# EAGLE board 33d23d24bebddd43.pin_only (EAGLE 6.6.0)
REV: B

Size 60.33 x 22.86 mm. Coordinates in mm from the lower left corner, seen from the top.
Outline: 2.54,0 57.78,0 arc90 60.33,2.54 60.33,20.32 arc90 57.78,22.86 2.54,22.86 arc90 0,20.32 0,14.1 0.51,13.59 0.51,9.4 0,8.89 0,2.54 arc90 2.54,0
Copper layers (1*16): Top 0.035mm / dielectric 1.5mm / Bottom 0.035mm
Design rules "adafruit 6-6 *": minimum track width 6mil, minimum drill 15.5mil, track to track 8mil, track to pad 6mil, pad to pad 8mil, via to via 8mil, smd to smd 8mil, copper to edge 10mil, drill to drill 8mil, minimum pad ring 10mil, minimum via ring 8mil, stop-mask expansion 2mil, vias tented up to drill 20mil, thermal gap 10mil
Holes 2.2 mm at 57.78,20.32
tRestrict: area 23.5,8.1 to 26.4,8.6; area 26.3,8.6 to 26.5,9.9; area 26.3,10.3 to 26.5,13.5; area 21,13.6 to 25.9,14; area 20.8,9.3 to 21.2,12.8; area 21.1,8.1 to 23,8.6; area 20.8,8.4 to 21.2,8.9; area 20.8,13.3 to 21.2,13.7

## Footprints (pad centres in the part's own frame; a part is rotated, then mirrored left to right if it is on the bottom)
_0805MP = smd 1.2 x 1.3: 1 -1.016,0; 2 1.016,0
0805-NO = smd 1.3 x 1.5: 1 -0.95,0; 2 0.95,0
C1210 = smd 1.6 x 2.7: 1 -1.4,0; 2 1.4,0
0603-NO = smd 1.1 x 1: 1 -0.85,0; 2 0.85,0
CHIPLED_0805_NOOUTLINE = smd 1.2 x 1.2: A 0,-1.05; C 0,1.05
SOD-323 = smd 1.35 x 0.8: A 1.27,0; C -1.27,0
SOT363 = smd 0.5 x 0.5: 1 -0.75,-0.9; 3 0.75,-0.9; 4 0.75,0.9; 6 -0.75,0.9 | smd 0.4 x 0.5: 2 0,-0.9; 5 0,0.9
SOD-123 = smd 1.4 x 1.4: A 1.85,0; C -1.85,0
TQFN44_7MM = smd 0.25 x 0.8: 1 -2.5,-3.475; 2 -2,-3.475; 3 -1.5,-3.475; 4 -1,-3.475; 5 -0.5,-3.475; 6 0,-3.475; 7 0.5,-3.475; 8 1,-3.475; 9 1.5,-3.475; 10 2,-3.475; 11 2.5,-3.475; 23 2.5,3.475; 24 2,3.475; 25 1.5,3.475; 26 1,3.475; 27 0.5,3.475; 28 0,3.475; 29 -0.5,3.475; 30 -1,3.475; 31 -1.5,3.475; 32 -2,3.475; 33 -2.5,3.475 | smd 0.8 x 0.25: 12 3.475,-2.5; 13 3.475,-2; 14 3.475,-1.5; 15 3.475,-1; 16 3.475,-0.5; 17 3.475,0; 18 3.475,0.5; 19 3.475,1; 20 3.475,1.5; 21 3.475,2; 22 3.475,2.5; 34 -3.475,2.5; 35 -3.475,2; 36 -3.475,1.5; 37 -3.475,1; 38 -3.475,0.5; 39 -3.475,0; 40 -3.475,-0.5; 41 -3.475,-1; 42 -3.475,-1.5; 43 -3.475,-2; 44 -3.475,-2.5 | smd 4.7 x 4.7: THERMAL 0,0
1X16_ROUND = drill 1 pad 1.676: 1 -19.05,0; 2 -16.51,0; 3 -13.97,0; 4 -11.43,0; 5 -8.89,0; 6 -6.35,0; 7 -3.81,0; 8 -1.27,0; 9 1.27,0; 10 3.81,0; 11 6.35,0; 12 8.89,0; 13 11.43,0; 14 13.97,0; 15 16.51,0; 16 19.05,0
1X12_ROUND = drill 1 pad 1.676: 1 -13.97,0; 2 -11.43,0; 3 -8.89,0; 4 -6.35,0; 5 -3.81,0; 6 -1.27,0; 7 1.27,0; 8 3.81,0; 9 6.35,0; 10 8.89,0; 11 11.43,0; 12 13.97,0
SOLDERJUMPER_CLOSEDWIRE = smd 1.168 x 1.6: 1 -0.762,0; 2 0.762,0 | smd 0.635 x 0.203: WIRE 0,0
KMR2 = smd 1 x 1: 1 2,0.8; 2 2,-0.8; 3 -2,0.8; 4 -2,-0.8
TESTPOINT_ROUND_1.5MM = smd 1.5 x 1.5: P$1 0,0
SIM800L = smd 1.1 x 0.9: 1 -8.1,5.6; 2 -8.1,4.2; 3 -8.1,2.8; 4 -8.1,1.4; 5 -8.1,0; 6 -8.1,-1.4; 7 -8.1,-2.8; 8 -8.1,-4.2; 9 -8.1,-5.6; 22 8.1,-5.6; 23 8.1,-4.2; 24 8.1,-2.8; 25 8.1,-1.4; 26 8.1,0; 27 8.1,1.4; 28 8.1,2.8; 29 8.1,4.2; 30 8.1,5.6; 43 -6.36,5.6; 44 -6.36,4.2; 45 -6.36,2.8; 46 -6.36,1.4; 47 -6.36,0; 48 -6.36,-1.4; 49 -6.36,-2.8; 50 -6.36,-4.2; 51 -6.36,-5.6; 60 6.36,-5.6; 61 6.36,-4.2; 62 6.36,-2.8; 63 6.36,-1.4; 64 6.36,0; 65 6.36,1.4; 66 6.36,2.8; 67 6.36,4.2; 68 6.36,5.6 | smd 0.9 x 1.1: 10 -7.7,-7.1; 11 -6.3,-7.1; 12 -4.9,-7.1; 13 -3.5,-7.1; 14 -2.1,-7.1; 15 -0.7,-7.1; 16 0.7,-7.1; 17 2.1,-7.1; 18 3.5,-7.1; 19 4.9,-7.1; 20 6.3,-7.1; 21 7.7,-7.1; 31 7.7,7.1; 32 6.3,7.1; 33 4.9,7.1; 34 3.5,7.1; 35 2.1,7.1; 36 0.7,7.1; 37 -0.7,7.1; 38 -2.1,7.1; 39 -3.5,7.1; 40 -4.9,7.1; 41 -6.3,7.1; 42 -7.7,7.1; 52 -4.9,-5.5; 53 -3.5,-5.5; 54 -2.1,-5.5; 55 -0.7,-5.5; 56 0.7,-5.5; 57 2.1,-5.5; 58 3.5,-5.5; 59 4.9,-5.5; 69 4.9,5.5; 70 3.5,5.5; 71 2.1,5.5; 72 0.7,5.5; 73 -0.7,5.5; 74 -2.1,5.5; 75 -3.5,5.5; 76 -4.9,5.5 | smd 1.5 x 1.5: 77 -3.9,3 | smd 2.3 x 2.7: 78 -3.9,0; 79 -3.9,-3; 80 -1.3,-3; 81 1.3,-3; 82 3.9,-3; 83 3.9,0; 84 3.9,3; 85 1.3,3; 86 -1.3,3; 87 -1.3,0; 88 1.3,0
SOT23-5 = smd 0.55 x 1.2: 1 -0.95,-1.3; 2 0,-1.3; 3 0.95,-1.3; 4 0.95,1.3; 5 -0.95,1.3
FIDUCIAL_1MM = smd 1 x 1: 1 0,0
MOUNTINGHOLE_2.5_PLATED = drill 2.5 pad 3.2: P$1 0,0
JSTPH2 = smd 1 x 4.6: 1 -1,-3.7; 2 1,-3.7 | smd 1.6 x 3.4: NC1 -3.4,1.5; NC2 3.4,1.5
4UCONN_20217 = smd 0.75 x 1.7: CLK -12.31,16.86; GND -5.96,16.86; I/O -11.04,16.86; RST -9.77,16.86; SW -4.69,16.86; VCC -7.23,16.86; VPP -8.5,16.86 | smd 1.4 x 1.05: GND@1 -15.53,17.06; GND@4 -0.33,17.06 | smd 1.5 x 2.7: GND@2 -15.86,1.42; GND@3 0,0
4UCONN_20329_V2 = smd 1 x 2: BASE@1 -0.75,-2; BASE@2 0.75,-2 | smd 0.4 x 1.35: D+ 0,0.775; D- -0.65,0.775; GND 1.3,0.775; ID 0.65,0.775; VBUS -1.3,0.775 | drill 0.8 pad 1.2 offset: SPRT@1 -3.3,0.9; SPRT@2 3.3,0.9 | drill 0.9 pad 2.5 square: SPRT@3 -3.6,-1.9; SPRT@4 3.6,-1.9 | hole 0.7: -1.95,0; 1.95,0
U.FL = smd 2.2 x 1.05: 1 0,1.375; 2 0,-1.375 | smd 0.8 x 1: 3 1.525,0
87758-0216 = drill 0.9 pad 1.27: 1 0,-1; 2 0,1
ANT_2450AT18B100 = smd 1.6 x 1.8: FP -1.4,0; NC 1.4,0
RESONATOR-SMD = smd 0.7 x 1.7: 1 -1.2,0; 2 0,0; 3 1.2,0

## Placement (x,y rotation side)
C1  10uF  [_0805MP]  37.27,9.02 180 top
C2  33pF  [0805-NO]  53.59,21.59 0 top
C3  10µF  [0805-NO]  11.81,12.06 0 top
C4  100uF  [C1210]  36.2,5.71 0 top
C5  10pF  [0805-NO]  50.16,21.59 180 top
C6  10µF  [0805-NO]  8.09,12.96 90 top
C7  1uF  [0603-NO]  18.94,15.04 90 top
C8  10µF  [0805-NO]  14.37,11.62 270 top
C9  10uF  [_0805MP]  29.57,15.46 180 top
C14  1uF  [0603-NO]  10.72,4.22 0 top
CHG  ORANGE  [CHIPLED_0805_NOOUTLINE]  2.41,5.59 270 top
D1  1N4148  [SOD-323]  33.78,12.32 270 top
D2  SMF05C  [SOT363]  37.47,12.19 0 top
D3  1N4148  [SOD-323]  32.77,17.4 270 top
D4  MBR120  [SOD-123]  17.91,18.92 180 top
D5  MMSZ5231BT1G  [SOD-123]  32.51,7.11 90 top
D7  1N4148  [SOD-323]  48.39,1.52 0 top
D9  1N4148  [SOD-323]  54.99,1.52 0 top
IC1  ATMEGA32U4-MU  [TQFN44_7MM]  23.72,11.1 0 top
JP1  [1X16_ROUND]  25.4,1.27 180 top
JP3  [1X12_ROUND]  30.48,21.59 0 top
L  RED  [CHIPLED_0805_NOOUTLINE]  2.65,17.36 90 top
NETSTAT  BLUE  [CHIPLED_0805_NOOUTLINE]  58.29,4.83 90 top
PWRSTAT  GREEN  [CHIPLED_0805_NOOUTLINE]  58.29,7.75 90 top
R1  1K  [0603-NO]  58.29,9.14 180 top
R2  1K  [0603-NO]  6.22,4.19 0 top
R3  1K  [0603-NO]  58.29,3.43 180 top
R4  22  [0603-NO]  8.22,10.27 0 top
R5  22  [0603-NO]  8.15,8.88 0 top
R6  100k  [0603-NO]  17.4,17.42 0 top
R7  2.2K  [0603-NO]  5.71,20.95 270 top
R8  2.2K  [0603-NO]  13.84,4.19 180 top
R9  DNP  [0603-NO]  32.38,12.06 90 top
SJ1  [SOLDERJUMPER_CLOSEDWIRE]  48.51,1.14 0 bottom
SW1  SPST_TACT-KMR2  [KMR2]  9.4,6.48 180 top
TP1  [TESTPOINT_ROUND_1.5MM]  37.34,8.76 0 bottom
U1  SIM800H/L  [SIM800L]  47.12,11.43 270 top
U2  AP2112-3.3K  [SOT23-5]  16.56,14.81 180 top
U3  MCP73831T-2ACI/OT  [SOT23-5]  13.97,7.75 180 top
U$7  [ADAFRUIT_3.5MM]  15.88,5.84 0 top
U$18  FIDUCIAL""  [FIDUCIAL_1MM]  9.27,6.35 0 top
U$23  FIDUCIAL""  [FIDUCIAL_1MM]  3.68,17.65 0 bottom
U$25  [FEATHERLOGO]  30.73,4.19 0 bottom
U$31  MOUNTINGHOLE2.5  [MOUNTINGHOLE_2.5_PLATED]  2.54,20.32 270 top
U$32  MOUNTINGHOLE2.5  [MOUNTINGHOLE_2.5_PLATED]  2.54,2.54 270 top
U$34  FIDUCIAL""  [FIDUCIAL_1MM]  10.79,20.07 270 top
U$35  FIDUCIAL""  [FIDUCIAL_1MM]  46.28,22.11 270 top
U$42  FIDUCIAL""  [FIDUCIAL_1MM]  54.36,0.76 0 bottom
U$43  [FONA_LOGO_SMALL]  30.23,10.54 0 bottom
U$44  [PCBFEAT-REV-040]  17.53,11.18 0 top
X1  JSTPH  [JSTPH2]  10.79,19.3 0 top
X2  4UCON 20217  [4UCONN_20217]  56.64,3.56 270 bottom
X3  microUSB  [4UCONN_20329_V2]  4.45,11.43 270 top
X4  uFL  [U.FL]  57.66,16.38 180 top
X5  1x2  [87758-0216]  36.58,17.14 270 top
X6  1x2  [87758-0216]  36.58,15.11 270 top
X7  ANT_2450AT18B100  [ANT_2450AT18B100]  57.78,11.18 0 top
Y1  8MHz  [RESONATOR-SMD]  28.37,5.26 180 top

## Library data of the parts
C1-C3 C5-C7 C9 C14 CHG D1-D5 D7 D9 IC1 JP1 JP3 L NETSTAT PWRSTAT R1-R9 SJ1 TP1 U1-U3 U$7 U$25 U$43 U$44 X1-X4 X7 = microbuilder
C4 = rcl
C8 = microbuilder; COMPANY: ADAFRUIT INDUSTRIES; DRAWN: KTOWN; REV: A
SW1 = adafruit
U$18 U$23 U$31 U$32 U$34 U$35 U$42 = microbuilder; BOM: EXCLUDE
X5 X6 = con-molex; MPN: 87758-0216; OC_FARNELL: unknown; OC_NEWARK: 94M1513
Y1 = SparkFun

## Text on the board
tPlace: 3 | 2 | BAT | En | USB | 13 | 12 | 11 | 10 | ~ | 9 | 6 | 5 | ~ | ~ | +mic- | #13 | Feather 32u4 | FONA | spk | + - | RST | adafruit! | PWR | NET | CHG | A0 | A1 | A2 | A3 | A4 | A5 | SCK | RST | 3V | ARf | GND | MO / SI | MI / SO | 0 | 1 | Key
bPlace: 3 | 2 | 2 | 3.7/4.2V / LiPoly Batt / µUSB charge | SDA | BAT | USB | 6 | ~ | 5 | En | 13 | 12 | 11~ | 10~ | 9~ | -mic+ | Feather 32u4 / FONA GSM | -spk+ | ATmega32u4 / 8MHz & 3.3V | 2G MicroSIM | FM / ANT | MOSI | MISO | RST | 3V | ARf | GND | A0 | A1 | A2 | A3 | A4 | A5 | SCK | RX | TX | KEY | 0 | 0 | 1 | 1

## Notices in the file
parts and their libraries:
microbuilder: This work is placed in the public domain, and may be freely used for commercial and non-commercial work with the following conditions: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
SparkFun: Licensing: CC v3.0 Share-Alike You are welcome to use this library for commercial purposes.
